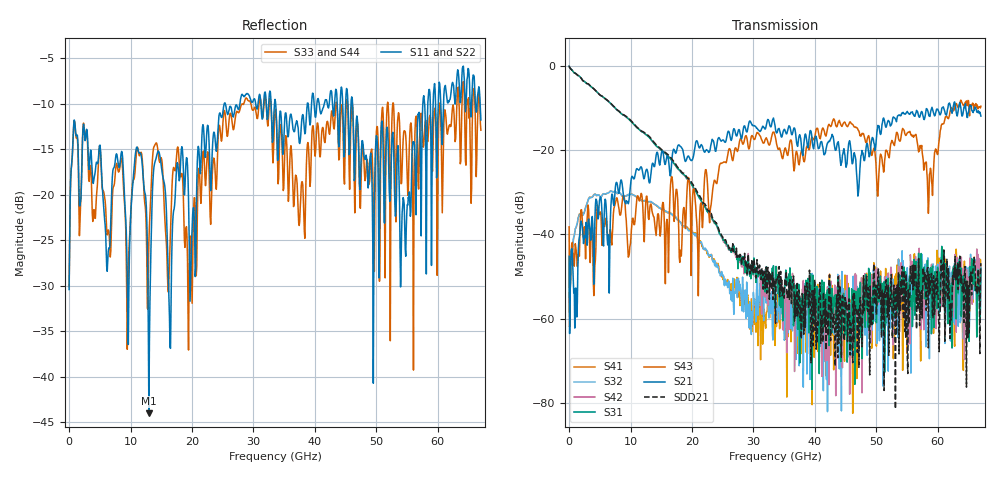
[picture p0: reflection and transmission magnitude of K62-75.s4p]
!Agilent Technologies,N5247A,US50470101,A.10.25.02
!Agilent N5247A: A.10.25.02
!Date: Tuesday, May 12, 2015 13:45:04
!Correction: Sdd11(Full 4 Port(1,2,3,4))
!Sdc11(Full 4 Port(1,2,3,4))
!Sdd12(Full 4 Port(1,2,3,4))
!Sdc12(Full 4 Port(1,2,3,4))
!Scd11(Full 4 Port(1,2,3,4))
!Scc11(Full 4 Port(1,2,3,4))
!Scd12(Full 4 Port(1,2,3,4))
!Scc12(Full 4 Port(1,2,3,4))
!Sdd21(Full 4 Port(1,2,3,4))
!Sdc21(Full 4 Port(1,2,3,4))
!Sdd22(Full 4 Port(1,2,3,4))
!Sdc22(Full 4 Port(1,2,3,4))
!Scd21(Full 4 Port(1,2,3,4))
!Scc21(Full 4 Port(1,2,3,4))
!Scd22(Full 4 Port(1,2,3,4))
!Scc22(Full 4 Port(1,2,3,4))
!Balanced Topology: BBAL
!S4P File: Measurements: <Sdd11,Sdc11,Sdd12,Sdc12>,
!<Scd11,Scc11,Scd12,Scc12>,
!<Sdd21,Sdc21,Sdd22,Sdc22>,
!<Scd21,Scc21,Scd22,Scc22>:
# Hz S  dB  R 50
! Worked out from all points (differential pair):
!   801 points, 10 MHz to 67 GHz, reference 50 ohm
!   strongest paths, dB at 10 MHz, 16.76 GHz, 33.51 GHz, 50.25 GHz, 67 GHz:
!     S21: -45.2, -21.8, -14.2, -14.2, -12.0
!     S43: -38.2, -26.4, -16.6, -30.9, -9.6
!     S31: -0.1, -22.6, -57.5, -51.0, -48.1
!     S42: -0.1, -22.6, -50.9, -56.7, -48.1
!     S32: -50.7, -35.4, -56.7, -55.2, -47.8
!     S41: -54.0, -35.3, -66.4, -55.6, -48.5
!   taken as a pair (ports 1,2 in; 3,4 out), SDD21 dB: -0.1, -22.2, -52.7, -49.1, -46.9
!   lowest |S11| = -44.0 dB at 12.99 GHz (marker M1), VSWR 1.01, Z = 50.1 - j0.621 ohm
!   |S11| at or under -10 dB: start of sweep to 25.25 GHz; 33.61 GHz to 38.77 GHz (5.156 GHz wide, 14.2 % of centre); 46.12 GHz to 57.56 GHz (11.44 GHz wide, 22.1 % of centre)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
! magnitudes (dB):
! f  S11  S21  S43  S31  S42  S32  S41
! 10 MHz  -30.4  -45.2  -38.2  -0.1  -0.1  -50.7  -54.0
! 3.36 GHz  -16.4  -38.3  -44.0  -4.7  -4.7  -31.2  -31.2
! 12.99 GHz  -44.0  -27.5  -36.5  -16.9  -16.9  -32.3  -32.3
! 14.41 GHz  -15.3  -20.7  -35.2  -19.3  -19.3  -33.3  -33.5
! 37.36 GHz  -13.4  -17.2  -23.4  -51.9  -52.8  -61.5  -67.4
! 58.71 GHz  -8.8  -12.0  -25.4  -50.1  -48.2  -52.5  -48.7
! 67 GHz  -11.8  -12.0  -9.6  -48.1  -48.1  -47.8  -48.5
